(* Logix 5000 AddOnInstructionDefinition export TorchWizard_Ethernet_Reamer; software revision 23.00 *)

ADD_ON_INSTRUCTION TorchWizard_Ethernet_Reamer   (* revision 2.1 *)
// Revision note:
// Revision 2.1 - Fixed Wire Cut operation
VAR_OUTPUT
   READY : BOOL; {visible}
END_VAR
VAR_IN_OUT
   INPUT_DATA : INT[16]; {required}
   OUTPUT_DATA : INT[16]; {required}
END_VAR
VAR_INPUT
   START_AUTO_SEQUENCE : BOOL; {visible}   // Start TorchWizard with all selected features and timer settings
   START_AUTO_SPRAY : BOOL; {visible}   // Start Anti-Spatter Sprayer after Torch Wizard REQ ACK
   START_AUTO_CUT : BOOL; {visible}   // Start Wire Cutter after TorchWizard REQ ACK
   ERROR_RETRY : BOOL; {visible}   // Acknowledge error message and restart machine at step immediately piror to where the error took place
   ERROR_IGNORE : BOOL; {visible}   // Acknowledge error message and continue to the next sequence step
   RESET_SEQUENCE_TIMERS : BOOL;   // Reset Timer Values to Default
   ENABLE_SPATTER_BREAK : BOOL;   // Optional Feature: Turn on the Spatter Break option
   ENABLE_WIRE_CUTTER : BOOL;   // Optional Feature: Turn on the Wire Cutter Feature at the end of the sequence
   ENABLE_GAS_FLOW_CHECK : BOOL;   // Optional Feature: Check Gas Flow prior to applying anti-spatter
   ENABLE_AIR_BLAST : BOOL;   // Optional Feature: Enable Self Cleaning Air Blast after Ream Cycle
   ENABLE_POST_REAM_NOZZLE_CHECK : BOOL;   // Optional Feature: Check Nozzle Prox Switch post Ream Cycle
   ENABLE_PRE_REAM_NOZZLE_CHECK : BOOL;   // Optional Feature: Check Nozzle Prox Switch pre Ream cycle
   CUSTOM_SPATTER_BREAK_SEQ_TIME : INT;
   CUSTOM_REAM_SEQ_TIME : INT;
   CUSTOM_AIR_BLAST_TIME : INT;
   CUSTOM_ANTI_SPATTER_SEQ_TIME : INT;
END_VAR
VAR_OUTPUT
   READY_TO_SPRAY : BOOL; {access None, visible}   // TorchWizard is ready to apply Anti-Spatter Spray
   READY_TO_CUT : BOOL; {access None, visible}   // TorchWizard is ready to run the Wire Cutter
   ERROR_ACTIVE : BOOL; {visible}
   REQUEST_ERROR_ACK : BOOL; {access None, visible}   // Torch Wizard is in the fault state and waiting for acknowledgement
   CURRENT_PROGRAM_STATE : INT; {access None}   // 0 IDLE, 1 ERROR ACTIVE, 2 ERROR MISSING NOZZLE, 3 ERROR CLAMP OPEN, 4 ERROR CLAMP CLOSED, 5 ERROR SLIDE UP, 6 ERROR SLIDE DOWN, 7 ERROR PREREAM NOZZLE CHECK, 8 ERROR POSTREAM NOZZLE CHECK, 9 ERROR GAS FLOW CHECK, 10 WAITING FOR NOZZLE, 11 WAITING FOR SLIDE DOWN, 12 WAITING FOR CLAMP CLOSE, 13 WAITING FOR CLAMP OPEN, 14 WAITING FOR NOZZLE TO CLEAR, 15 WAITING FOR REAM ACK, 16 WAITING FOR SPRAY ACK, 17 WAITING FOR CUT ACK, 18 WAITING FOR SPRAY DELAY TIMER, 19 WAITING FOR REAM DELAY TIMER, 20 WAITING FOR CUT D
   PREVIOUS_CYCLE_TIME : DINT; {access None, visible}   // Previous Cycle Time in milliseconds
   ERROR_01_PRE_REAM_NC : BOOL; {access None, visible}
   ERROR_02_CLAMP_STUCK_IN_HOME : BOOL; {access None, visible}
   ERROR_03_NOZZLE_NOT_PRESENT : BOOL; {access None, visible}
   ERROR_04_SLIDE_STUCK_UP_SPATTER_BREAK : BOOL; {access None, visible}
   ERROR_05_SLIDE_STUCK_UP_REAMING_CYCLE : BOOL; {access None, visible}
   ERROR_06_NOZZLE_PRESENT : BOOL; {access None, visible}
   ERROR_07_CLAMP_NOT_IN_HOME : BOOL; {access None, visible}
   ERROR_08_POST_REAM_NOZZLE_CHECK : BOOL; {access None, visible}
   ERROR_09_GAS_FLOW_CHECK : BOOL; {access None, visible}
   SPATTER_BREAK_ENABLED : BOOL; {access None, visible}   // Enabled Setting Feedback from TorchWizard
   WIRE_CUTTER_ENABLED : BOOL; {access None, visible}   // Enabled Setting Feedback from TorchWizard
   GAS_FLOW_CHECK_ENABLED : BOOL; {access Read Only, visible}   // Enabled Setting Feedback from TorchWizard
   SELF_CLEAN_AIR_BLAST_ENABLED : BOOL; {access None, visible}   // Enabled Setting Feedback from TorchWizard
   POST_REAM_NC_ENABLED : BOOL; {access None, visible}   // Enabled Setting Feedback from TorchWizard
   PRE_REAM_NC_ENABLED : BOOL; {access None, visible}   // Enabled Setting Feedback from TorchWizard
   SEQUENCE_COMPLETE : BOOL; {visible}
END_VAR
VAR_INPUT
   ENABLE_SEMI_AUTO_MODE : BOOL; {visible}
   SEMI_AUTO_REAM : BOOL; {visible}
   SEMI_AUTO_SPRAY : BOOL; {visible}
   SEMI_AUTO_SELF_CLEAN_AIR_BLAST : BOOL; {visible}
   SEMI_AUTO_WIRECUT : BOOL; {visible}
   DISABLE_DIAGNOSTICS : BOOL;
   RESET : BOOL; {visible}
END_VAR
VAR
   Start_Sequence_SB : BOOL; {access None}
   Start_Sequence_OB : BOOL; {access None}
   Stop_SB : BOOL; {access None}
   Stop_OB : BOOL; {access None}
   Er_Retry_SB : BOOL; {access None}
   Er_Retry_OB : BOOL; {access None}
   Er_Ignore_SB : BOOL; {access None}
   Er_Ignore_OB : BOOL; {access None}
   OSR_IGNORE_OB : BOOL; {access None}
   OSR_IGNORE_SB : BOOL; {access None}
   IOL_Master : INT; {access None}
        .0   // TURCK
        .1   // BALLUFF
        .2   // IFM
        .3   // Any IO-Link Master
   ons_start_bit : BOOL; {access None}
   ons_reset : BOOL; {access None}
END_VAR

ROUTINE Logic   (* ladder *)
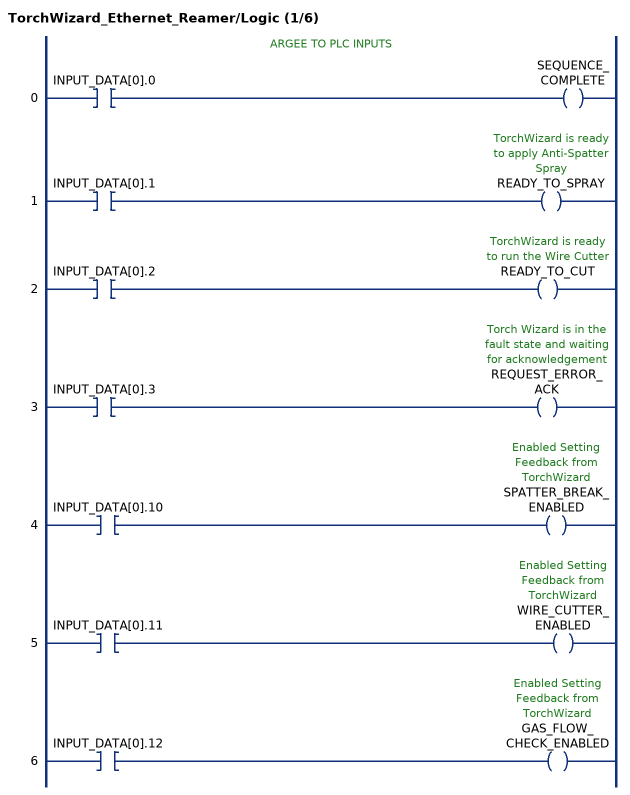
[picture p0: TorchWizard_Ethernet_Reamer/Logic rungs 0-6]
   // ARGEE TO PLC INPUTS
   0: XIC(INPUT_DATA[0].0)OTE(SEQUENCE_COMPLETE);
   1: XIC(INPUT_DATA[0].1)OTE(READY_TO_SPRAY);
   2: XIC(INPUT_DATA[0].2)OTE(READY_TO_CUT);
   3: XIC(INPUT_DATA[0].3)OTE(REQUEST_ERROR_ACK);
   4: XIC(INPUT_DATA[0].10)OTE(SPATTER_BREAK_ENABLED);
   5: XIC(INPUT_DATA[0].11)OTE(WIRE_CUTTER_ENABLED);
   6: XIC(INPUT_DATA[0].12)OTE(GAS_FLOW_CHECK_ENABLED);
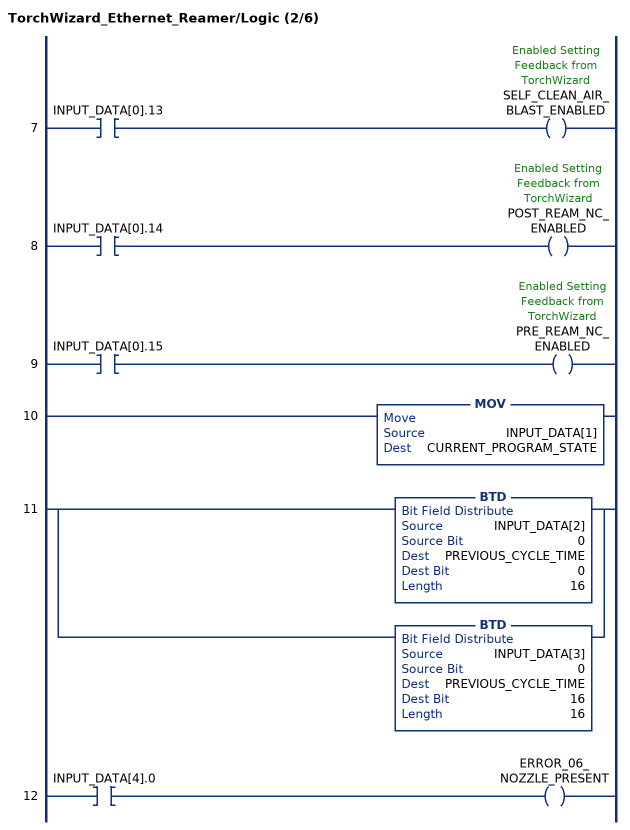
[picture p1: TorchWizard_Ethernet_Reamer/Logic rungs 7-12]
   7: XIC(INPUT_DATA[0].13)OTE(SELF_CLEAN_AIR_BLAST_ENABLED);
   8: XIC(INPUT_DATA[0].14)OTE(POST_REAM_NC_ENABLED);
   9: XIC(INPUT_DATA[0].15)OTE(PRE_REAM_NC_ENABLED);
   10: MOV(INPUT_DATA[1],CURRENT_PROGRAM_STATE);
   11: [BTD(INPUT_DATA[2],0,PREVIOUS_CYCLE_TIME,0,16) ,BTD(INPUT_DATA[3],0,PREVIOUS_CYCLE_TIME,16,16) ];
   12: XIC(INPUT_DATA[4].0)OTE(ERROR_06_NOZZLE_PRESENT);
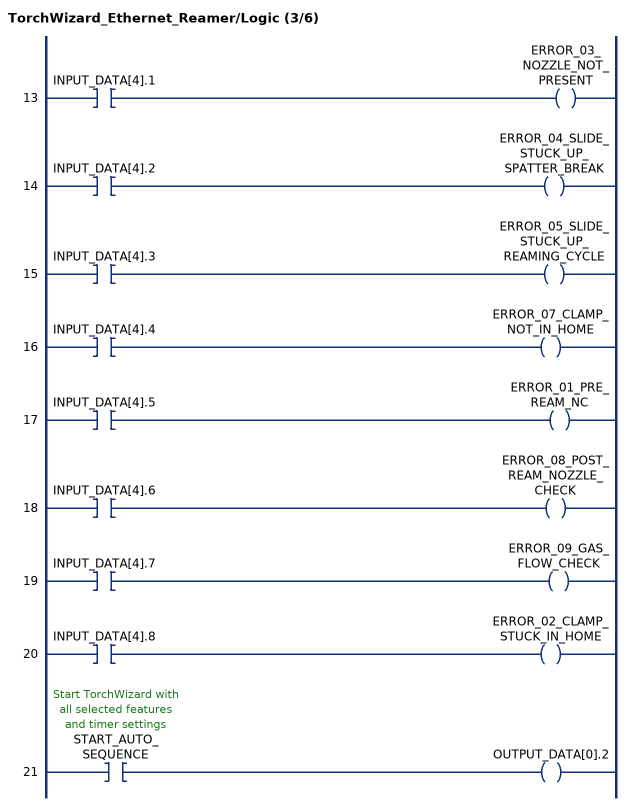
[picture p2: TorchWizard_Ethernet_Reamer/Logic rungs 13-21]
   13: XIC(INPUT_DATA[4].1)OTE(ERROR_03_NOZZLE_NOT_PRESENT);
   14: XIC(INPUT_DATA[4].2)OTE(ERROR_04_SLIDE_STUCK_UP_SPATTER_BREAK);
   15: XIC(INPUT_DATA[4].3)OTE(ERROR_05_SLIDE_STUCK_UP_REAMING_CYCLE);
   16: XIC(INPUT_DATA[4].4)OTE(ERROR_07_CLAMP_NOT_IN_HOME);
   17: XIC(INPUT_DATA[4].5)OTE(ERROR_01_PRE_REAM_NC);
   18: XIC(INPUT_DATA[4].6)OTE(ERROR_08_POST_REAM_NOZZLE_CHECK);
   19: XIC(INPUT_DATA[4].7)OTE(ERROR_09_GAS_FLOW_CHECK);
   20: XIC(INPUT_DATA[4].8)OTE(ERROR_02_CLAMP_STUCK_IN_HOME);
   21: XIC(START_AUTO_SEQUENCE)OTE(OUTPUT_DATA[0].2);
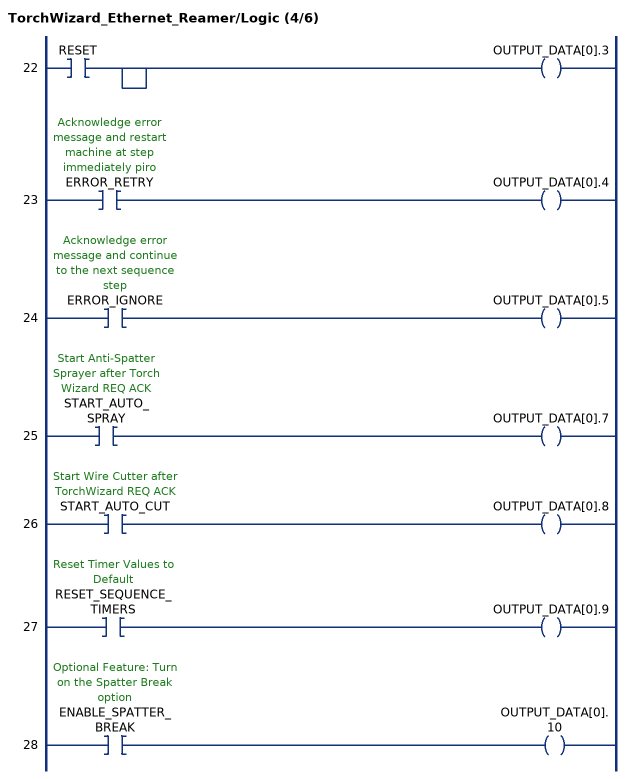
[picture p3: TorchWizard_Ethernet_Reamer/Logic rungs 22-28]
   22: XIC(RESET)[,]OTE(OUTPUT_DATA[0].3);
   23: XIC(ERROR_RETRY)OTE(OUTPUT_DATA[0].4);
   24: XIC(ERROR_IGNORE)OTE(OUTPUT_DATA[0].5);
   25: XIC(START_AUTO_SPRAY)OTE(OUTPUT_DATA[0].7);
   26: XIC(START_AUTO_CUT)OTE(OUTPUT_DATA[0].8);
   27: XIC(RESET_SEQUENCE_TIMERS)OTE(OUTPUT_DATA[0].9);
   28: XIC(ENABLE_SPATTER_BREAK)OTE(OUTPUT_DATA[0].10);
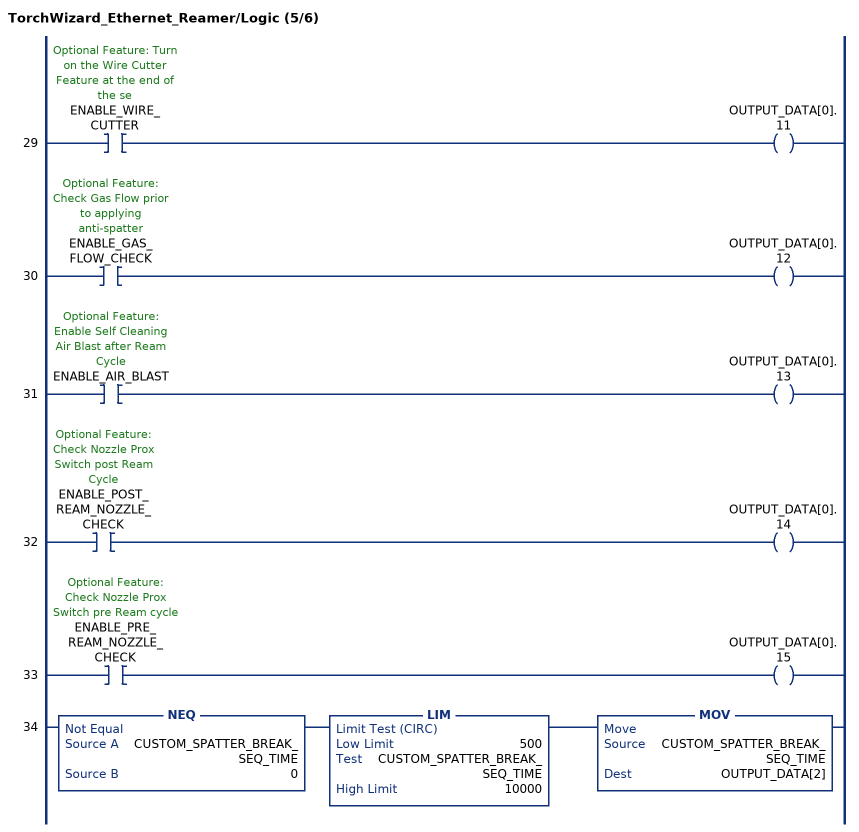
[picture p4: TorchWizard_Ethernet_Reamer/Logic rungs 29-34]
   29: XIC(ENABLE_WIRE_CUTTER)OTE(OUTPUT_DATA[0].11);
   30: XIC(ENABLE_GAS_FLOW_CHECK)OTE(OUTPUT_DATA[0].12);
   31: XIC(ENABLE_AIR_BLAST)OTE(OUTPUT_DATA[0].13);
   32: XIC(ENABLE_POST_REAM_NOZZLE_CHECK)OTE(OUTPUT_DATA[0].14);
   33: XIC(ENABLE_PRE_REAM_NOZZLE_CHECK)OTE(OUTPUT_DATA[0].15);
   34: NEQ(CUSTOM_SPATTER_BREAK_SEQ_TIME,0)LIM(500,CUSTOM_SPATTER_BREAK_SEQ_TIME,10000)MOV(CUSTOM_SPATTER_BREAK_SEQ_TIME,OUTPUT_DATA[2]);
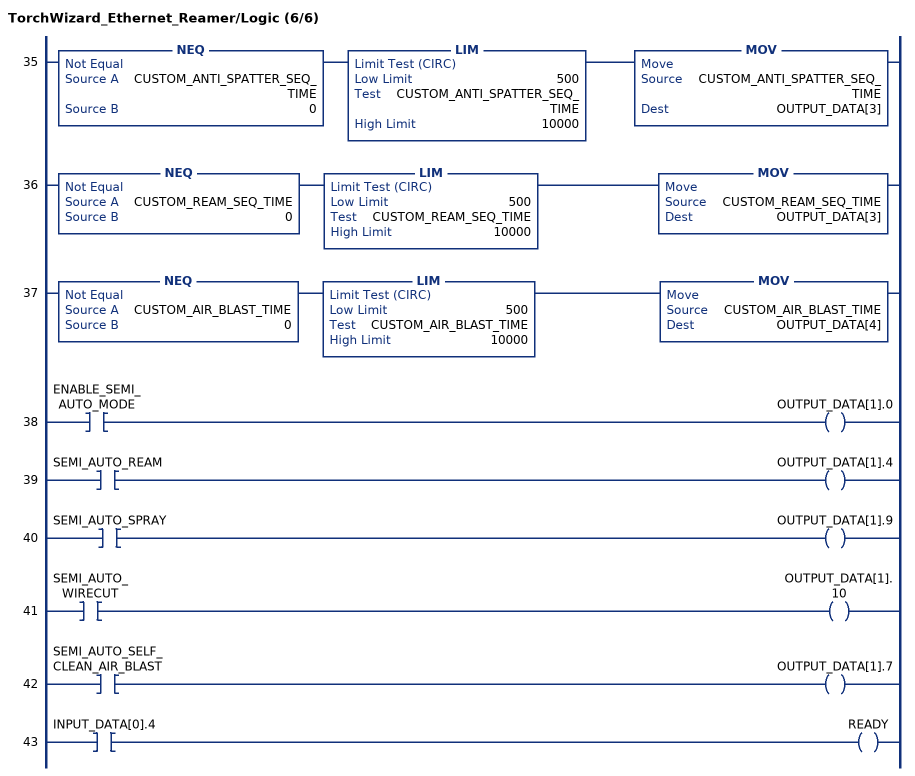
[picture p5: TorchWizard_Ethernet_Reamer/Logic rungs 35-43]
   35: NEQ(CUSTOM_ANTI_SPATTER_SEQ_TIME,0)LIM(500,CUSTOM_ANTI_SPATTER_SEQ_TIME,10000)MOV(CUSTOM_ANTI_SPATTER_SEQ_TIME,OUTPUT_DATA[3]);
   36: NEQ(CUSTOM_REAM_SEQ_TIME,0)LIM(500,CUSTOM_REAM_SEQ_TIME,10000)MOV(CUSTOM_REAM_SEQ_TIME,OUTPUT_DATA[3]);
   37: NEQ(CUSTOM_AIR_BLAST_TIME,0)LIM(500,CUSTOM_AIR_BLAST_TIME,10000)MOV(CUSTOM_AIR_BLAST_TIME,OUTPUT_DATA[4]);
   38: XIC(ENABLE_SEMI_AUTO_MODE)OTE(OUTPUT_DATA[1].0);
   39: XIC(SEMI_AUTO_REAM)OTE(OUTPUT_DATA[1].4);
   40: XIC(SEMI_AUTO_SPRAY)OTE(OUTPUT_DATA[1].9);
   41: XIC(SEMI_AUTO_WIRECUT)OTE(OUTPUT_DATA[1].10);
   42: XIC(SEMI_AUTO_SELF_CLEAN_AIR_BLAST)OTE(OUTPUT_DATA[1].7);
   43: XIC(INPUT_DATA[0].4)OTE(READY);
END_ROUTINE
END_ADD_ON_INSTRUCTION
